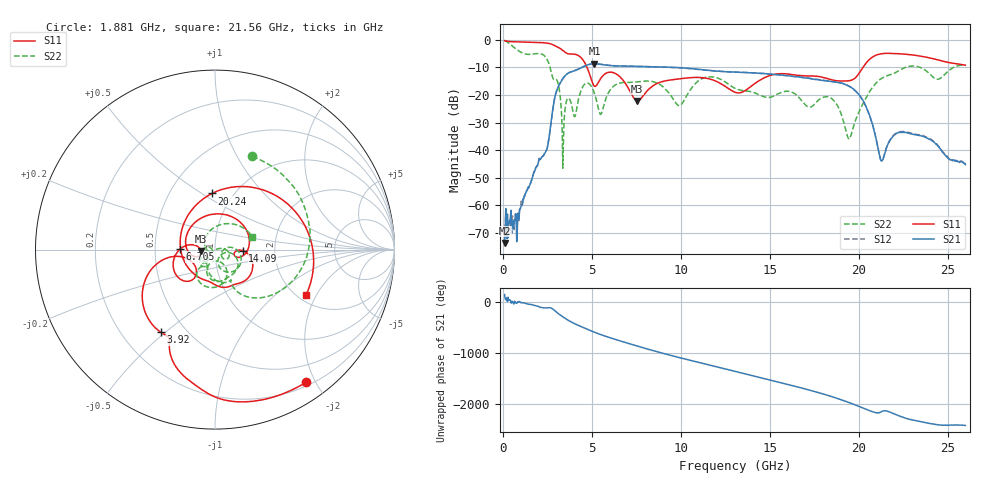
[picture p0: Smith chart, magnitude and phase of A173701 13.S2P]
!  2-Port S-parameters saved by WinCal
! VAR MeasName=S-Parameters (CALIBRATED_DATA) read from VNA (N5245A)
! VAR MeasDate=2017-6-7 10:29:15
! VAR NAME=A173701 13
! VAR FILENAME=A173701 13.S2P
! VAR DATE=2017-6-7 10:29:15
! VAR PHYS_PORTS=1,2
# Hz S DB R 50
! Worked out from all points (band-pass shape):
!   801 points, 100 MHz to 26 GHz, reference 50 ohm
!   highest |S21| = -8.70 dB at 5.151 GHz (marker M1); lowest = -73.6 dB at 100 MHz (marker M2)
!   |S21| within 3 dB of the highest: 3.814 GHz to 12.99 GHz (9.178 GHz wide, 109 % of centre)
!   lowest |S11| = -22.2 dB at 7.546 GHz (marker M3), VSWR 1.17, Z = 42.8 - j0.708 ohm
!   |S11| at or under -10 dB: 4.732 GHz to 20.25 GHz (15.51 GHz wide, 124 % of centre)
!   |S22| runs from -46.6 to -0.3 dB; largest |S21 - S12| = 0.0045
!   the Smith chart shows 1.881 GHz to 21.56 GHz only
!   S11 on the Smith chart (normalised r, x): 1.881 GHz: 0.25, -1.88; 3.92 GHz: 0.36, -0.48; 6.705 GHz: 0.68, +0.00; 14.09 GHz: 1.36, -0.02; 20.24 GHz: 0.80, +0.55; 21.56 GHz: 2.22, -1.65
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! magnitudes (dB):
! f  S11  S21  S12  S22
! 100 MHz  -0.3  -73.6  -74.8  -0.3
! 1.881 GHz  -0.9  -46.2  -46.1  -5.0
! 3.046 GHz  -2.5  -18.1  -18.1  -14.7
! 3.37 GHz  -3.9  -14.2  -14.1  -46.6
! 3.92 GHz  -5.2  -11.5  -11.4  -25.3
! 4.438 GHz  -6.8  -10.1  -10.0  -17.7
! 5.151 GHz  -16.8  -8.7  -8.7  -19.5
! 5.507 GHz  -14.0  -8.9  -8.9  -27.0
! 6.705 GHz  -14.3  -9.5  -9.5  -15.6
! 7.546 GHz  -22.2  -9.6  -9.6  -15.2
! 8.744 GHz  -15.6  -9.8  -9.9  -16.0
! 9.91 GHz  -14.2  -10.1  -10.2  -23.9
! 13.05 GHz  -19.0  -11.7  -11.7  -17.6
! 14.09 GHz  -16.2  -12.0  -12.0  -19.1
! 17.39 GHz  -13.1  -14.2  -14.1  -24.1
! 18.49 GHz  -14.5  -15.2  -15.1  -21.4
! 19.46 GHz  -14.9  -16.9  -16.8  -36.0
! 20.24 GHz  -10.1  -21.9  -22.1  -23.2
! 21.24 GHz  -5.1  -43.6  -43.5  -14.2
! 21.56 GHz  -4.9  -39.2  -39.0  -13.1
! 21.69 GHz  -4.9  -37.2  -37.2  -12.8
! 26 GHz  -9.2  -45.3  -45.0  -9.3
